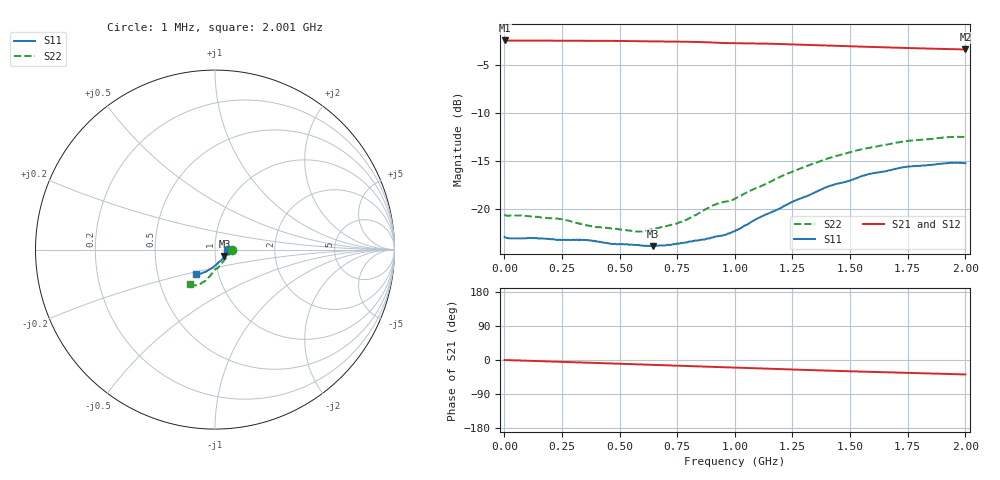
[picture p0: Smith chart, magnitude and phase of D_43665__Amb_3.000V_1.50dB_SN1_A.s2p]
! device id: 43665_
! dir: \\malibu\benchdata\1_engineers\tn_data\43665_75ohm\new\sparar\43665_\amb\3p000v\1p50db
! Serial: 1
! Insertion: A
! Temp: Amb
! VDD: 3.000V
! Attenuation Step: 1.50dB
! IDD: 1.451400e+00mA
! FILE NAME
! DATE 03-27-2009 08:33:44
! CORRECTED  DATA
#  Hz  S  RI  R  75
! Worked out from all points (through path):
!   401 points, 1 MHz to 2.001 GHz, reference 75 ohm
!   highest |S21| = -2.48 dB at 1 MHz (marker M1); lowest = -3.4 dB at 2.001 GHz (marker M2)
!   group delay of S21, straight-line fit = 54.1 ps
!   lowest |S11| = -23.8 dB at 646 MHz (marker M3), VSWR 1.14, Z = 83.1 - j6.12 ohm
!   |S11| at or under -10 dB: start of sweep to end of sweep
!   |S22| runs from -22.3 to -12.5 dB; largest |S21 - S12| = 0.0045
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1000000  0.0718 -0.00115  0.7516 -0.00121  0.7517 -0.00145  0.0939 -0.00148
2.36e8  0.0691 -0.00735  0.7474 -0.0596  0.7475 -0.06  0.0876 -0.0168
3.36e8  0.0682 -0.0124  0.744 -0.0853  0.7442 -0.0855  0.08 -0.0246
4.66e8  0.0628 -0.0203  0.738 -0.1186  0.7381 -0.1191  0.0693 -0.0386
5.76e8  0.058 -0.0298  0.7304 -0.1469  0.7304 -0.1473  0.0568 -0.0517
6.46e8  0.0529 -0.0367  0.7256 -0.1646  0.7253 -0.1651  0.0497 -0.0615
6.71e8  0.0515 -0.0395  0.7237 -0.171  0.7234 -0.1712  0.047 -0.0648
7.76e8  0.0424 -0.0518  0.7134 -0.1985  0.7133 -0.1986  0.0333 -0.0802
8.76e8  0.03 -0.0634  0.7007 -0.2242  0.7009 -0.2241  0.0189 -0.0985
9.31e8  0.0218 -0.0692  0.6913 -0.2361  0.6917 -0.2359  0.0082 -0.1073
9.56e8  0.0196 -0.0709  0.6879 -0.2401  0.6883 -0.2399  0.00269 -0.1093
1.001e9  0.0159 -0.0756  0.6843 -0.2487  0.6847 -0.2487  -0.00322 -0.1134
1.096e9  0.000764 -0.0893  0.6726 -0.2707  0.6733 -0.2709  -0.0131 -0.1284
1.211e9  -0.0167 -0.1022  0.656 -0.2964  0.657 -0.2971  -0.0281 -0.1473
1.336e9  -0.0369 -0.1147  0.6357 -0.3198  0.6367 -0.3208  -0.0467 -0.1653
1.406e9  -0.0487 -0.1219  0.624 -0.3335  0.625 -0.3352  -0.0551 -0.1754
1.491e9  -0.0609 -0.1258  0.6098 -0.3467  0.6102 -0.3486  -0.0704 -0.1832
1.566e9  -0.0727 -0.1317  0.5979 -0.3586  0.5981 -0.3613  -0.0804 -0.1901
1.671e9  -0.0849 -0.1348  0.5812 -0.3741  0.5801 -0.3767  -0.0966 -0.1952
1.756e9  -0.0933 -0.1382  0.5677 -0.3859  0.5665 -0.3888  -0.1082 -0.1995
1.931e9  -0.1052 -0.1386  0.5412 -0.4081  0.5394 -0.4092  -0.1333 -0.1958
2.001e9  -0.1065 -0.137  0.5311 -0.417  0.5271 -0.4189  -0.1411 -0.1908
